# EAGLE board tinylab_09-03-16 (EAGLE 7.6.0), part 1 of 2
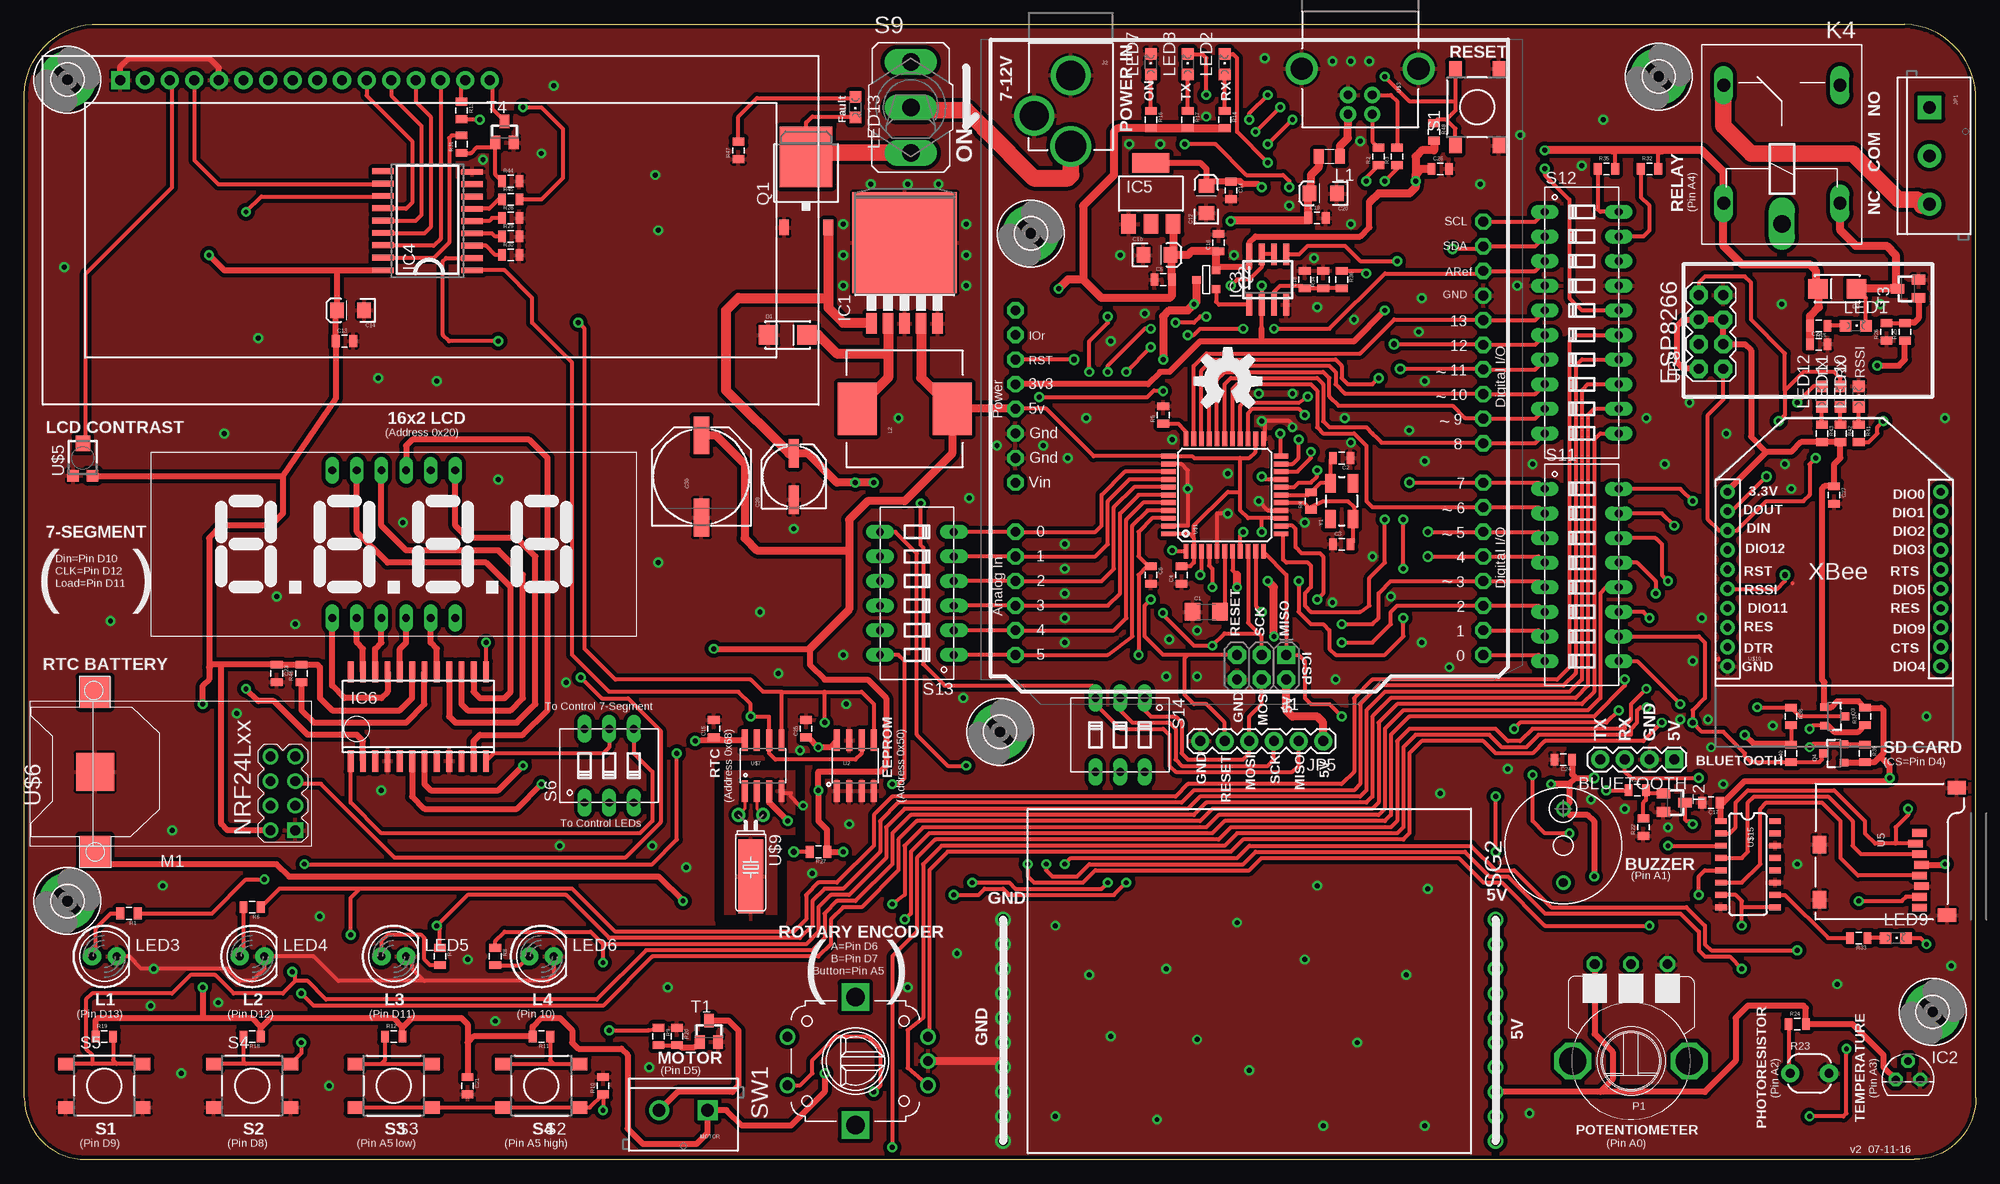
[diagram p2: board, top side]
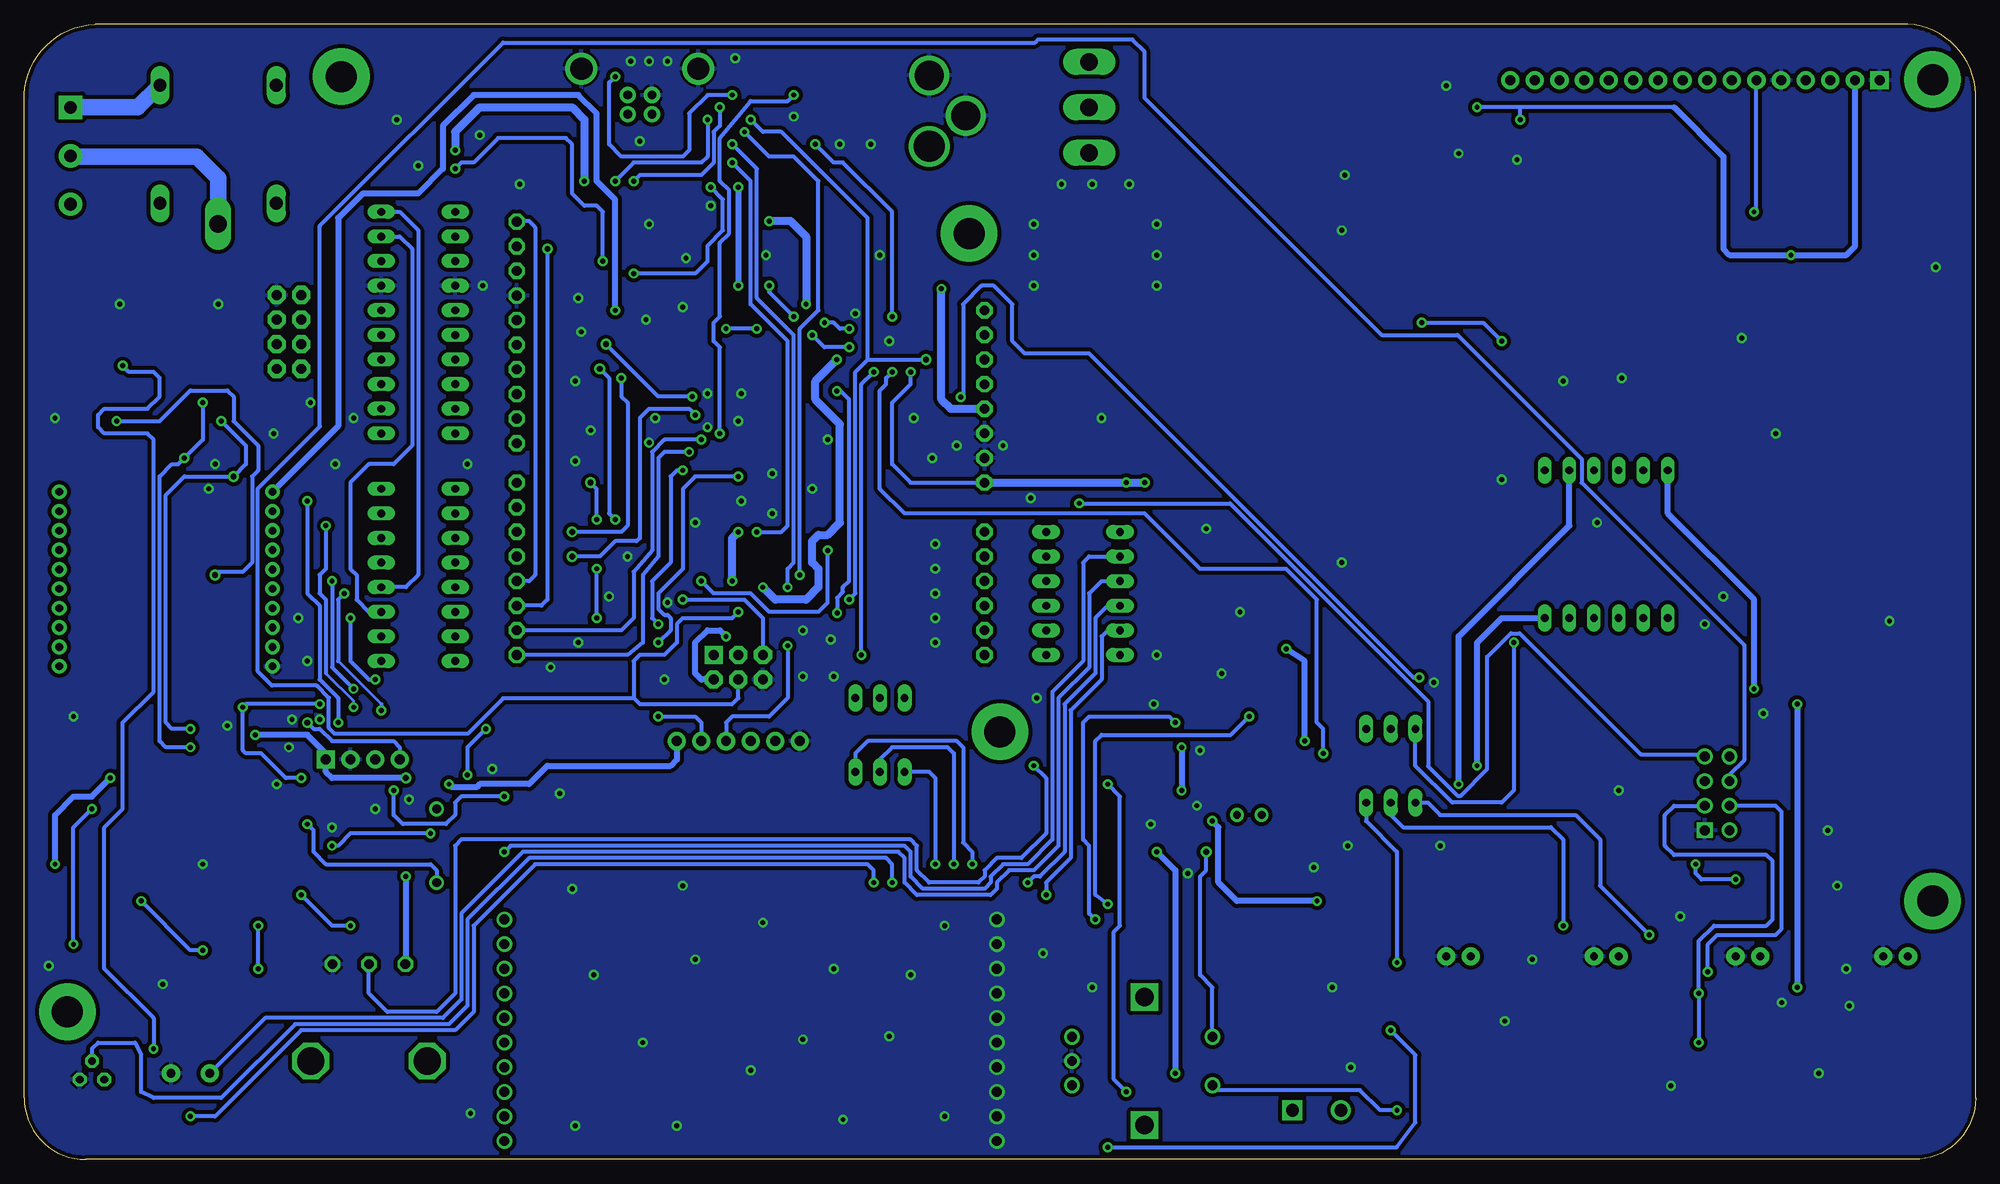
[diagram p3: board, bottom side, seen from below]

Size 201.31 x 117.16 mm. Coordinates in mm from the lower left corner, seen from the top.
Outline: 201.29,6.35 201.29,109.52
Outline: 201.31,6.35 arc-90 194.96,0 6.36,0 arc-90 0.01,6.35 0.01,109.22 arc-90 7,117.16 194,117.16 arc-90 201.31,109.22
Copper layers (1*16): Top 0.035mm / dielectric 1.5mm / Bottom 0.035mm
Design rules "default": minimum track width 16mil, minimum drill 20mil, track to track 8mil, track to pad 12mil, pad to pad 8mil, via to via 8mil, smd to smd 8mil, copper to edge 10mil, drill to drill 8mil, minimum pad ring 12mil, minimum via ring 10mil, stop-mask expansion 4mil, vias tented up to drill 25mil, thermal gap 10mil
tRestrict: 7 lines

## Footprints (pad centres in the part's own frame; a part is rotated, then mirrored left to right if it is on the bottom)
1X04 = drill 1.016 pad 1.88 square: 1 0,0 | drill 1.016 pad 1.88: 2 2.54,0; 3 5.08,0; 4 7.62,0
1206 = smd 1.6 x 1.8: 1 -1.4,0; 2 1.4,0
0805 = smd 0.8 x 1.2: 1 -0.9,0; 2 0.9,0
EIA3216 = smd 1.4 x 1.6: A 1.4,0; C -1.4,0
NIPPON_F80 = smd 2.95 x 1: + 2.4,0; - -2.4,0
PANASONIC_G = smd 3.9 x 1.6: + 4.25,0; - -4.25,0
SMA-DIODE_ALT = smd 2 x 2: A -2,0; C 2,0
3,2-PAD = drill 3.2 pad 5.842: B3,2 0,0
TO263-5 = smd 1.067 x 2.159: 1 -3.404,-5.791; 2 -1.702,-5.791; 3 0,-5.791; 4 1.702,-5.791; 5 3.404,-5.791 | smd 10.8 x 10.41: GND 0,2.54
TO92 = drill 0.813 octagon: 1 -1.27,0; 2 0,1.905; 3 1.27,0
SO08 = smd 0.6 x 2.2: 1 -1.905,-2.6; 2 -0.635,-2.6; 3 0.635,-2.6; 4 1.905,-2.6; 5 1.905,2.6; 6 0.635,2.6; 7 -0.635,2.6; 8 -1.905,2.6
SO18W = smd 0.6 x 2.2: 1 -4.445,-4.6; 2 -3.175,-4.6; 3 -1.905,-4.6; 4 -0.635,-4.6; 5 0.635,-4.6; 6 1.905,-4.6; 7 3.175,-4.6; 8 4.445,-4.6; 9 5.715,-4.6; 10 5.775,4.6; 11 4.505,4.6; 12 3.235,4.6; 13 1.965,4.6; 14 0.695,4.6; 15 -0.575,4.6; 16 -1.845,4.6; 17 -3.145,4.6; 18 -4.445,4.6
SOT223 = smd 1.5 x 2: 1 -2.3,-3.15; 2 0,-3.15; 3 2.3,-3.15 | smd 3.8 x 2: 4 0,3.15
SO24W = smd 0.6 x 2.2: 1 -6.985,-4.6; 2 -5.715,-4.6; 3 -4.445,-4.6; 4 -3.175,-4.6; 5 -1.905,-4.6; 6 -0.635,-4.6; 7 0.635,-4.6; 8 1.905,-4.6; 9 3.175,-4.6; 10 4.445,-4.6; 11 5.715,-4.6; 12 6.985,-4.6; 13 6.985,4.6; 14 5.715,4.6; 15 4.445,4.6; 16 3.175,4.6; 17 1.905,4.6; 18 0.635,4.6; 19 -0.635,4.6; 20 -1.905,4.6; 21 -3.175,4.6; 22 -4.445,4.6; 23 -5.715,4.6; 24 -6.985,4.6
2X3-NS = drill 1.016 pad 1.88 square: 1 -2.54,-1.27 | drill 1.016 pad 1.88 octagon: 2 -2.54,1.27; 3 0,-1.27; 4 0,1.27; 5 2.54,-1.27; 6 2.54,1.27
POWER_JACK_PTH_LOCK = drill 2.997 pad 4.115: GND 0.025,6.557; GNDBREAK 3.762,10.7 | drill 3.2 pad 4.115: PWR 0,13.878
SCREWTERMINAL-5MM-3 = drill 1.3 pad 2.413 square: 1 0,0 | drill 1.3 pad 2.413: 2 5,0; 3 10,0
1X06 = drill 1.016 pad 1.88: 1 0,0; 2 2.54,0; 3 5.08,0; 4 7.62,0; 5 10.16,0; 6 12.7,0
2X4 = drill 1.016 pad 1.88 octagon: 1 -3.81,-1.27; 2 -3.81,1.27; 3 -1.27,-1.27; 4 -1.27,1.27; 5 1.27,-1.27; 6 1.27,1.27; 7 3.81,-1.27; 8 3.81,1.27
ZF112 = drill 1.321 long: 1 -6.096,5.994; 2 -6.096,-5.994; O 6.096,5.994; S 6.096,-5.994 | drill 1.803 long: P -8.204,0
PTC0805 = smd 1 x 1.5: 1 -1.1,0; 2 1.1,0
CDRH125 = smd 5.4 x 4: 1 0,4.9; 2 0,-4.9
CHIPLED_0805 = smd 1.2 x 1.2: A 0,-1.05; C 0,1.05
LED5MM = drill 0.813 pad 1.88: A -1.27,0; K 1.27,0
WIRELESS-NRF24L01 = drill 1 square: 1 -12.7,6.35 | drill 1: 2 -10.16,6.35; 3 -12.7,3.81; 4 -10.16,3.81; 5 -12.7,1.27; 6 -10.16,1.27; 7 -12.7,-1.27; 8 -10.16,-1.27
SCREWTERMINAL-5MM-2 = drill 1.3 pad 2.032 square: 1 0,0 | drill 1.3 pad 2.032: 2 5,0
P120PK = drill 1 octagon: A -3.75,-10; E 3.75,-10; S 0,-10 | drill 2.8 octagon: M1 -6,0; M2 6,0
TO252 = smd 1 x 1.6: 1 -2.28,-4.8; 2 2.28,-4.8 | smd 5.4 x 6.2: 3 0,2.5
SOT-23 = smd 0.787 x 0.889: 1 0.025,-1.016; 2 -0.94,1.016; 3 0.991,1.016
SOT23-3 = smd 0.8 x 0.9: 1 -0.95,-1; 2 0.95,-1; 3 0,1.1
PHOTOCELL-KIT = drill 0.9 pad 1.88: 1 -2,0; 2 2,0
DTSM-6 = smd 1.55 x 1.3: 1 -3.975,2.25; 2 3.975,2.25; 3 -3.975,-2.25; 4 3.975,-2.25
DIP03YL = drill 0.813 long: 1 -2.54,-3.81; 2 0,-3.81; 3 2.54,-3.81; 4 2.54,3.81; 5 0,3.81; 6 -2.54,3.81
M9040P = drill 1.803 long: 1 0,4.699; 2 0,0; 3 0,-4.699
DIP08YL = drill 0.813 long: 1 -8.89,-3.81; 2 -6.35,-3.81; 3 -3.81,-3.81; 4 -1.27,-3.81; 5 1.27,-3.81; 6 3.81,-3.81; 7 6.35,-3.81; 8 8.89,-3.81; 9 8.89,3.81; 10 6.35,3.81; 11 3.81,3.81; 12 1.27,3.81; 13 -1.27,3.81; 14 -3.81,3.81; 15 -6.35,3.81; 16 -8.89,3.81
DIP10YL = drill 0.813 long: 1 -11.43,-3.81; 2 -8.89,-3.81; 3 -6.35,-3.81; 4 -3.81,-3.81; 5 -1.27,-3.81; 6 1.27,-3.81; 7 3.81,-3.81; 8 6.35,-3.81; 9 8.89,-3.81; 10 11.43,-3.81; 11 11.43,3.81; 12 8.89,3.81; 13 6.35,3.81; 14 3.81,3.81; 15 1.27,3.81; 16 -1.27,3.81; 17 -3.81,3.81; 18 -6.35,3.81; 19 -8.89,3.81; 20 -11.43,3.81
DIP06YL = drill 0.813 long: 1 -6.35,-3.81; 2 -3.81,-3.81; 3 -1.27,-3.81; 4 1.27,-3.81; 5 3.81,-3.81; 6 6.35,-3.81; 7 6.35,3.81; 8 3.81,3.81; 9 1.27,3.81; 10 -1.27,3.81; 11 -3.81,3.81; 12 -6.35,3.81
BMT1205XH7.5 = drill 0.9 pad 1.5: + 3.8,0; - -3.8,0
PEC12_INCREMENTAL_ENCODER = drill 1: A -2.5,-7.5; B 2.5,-7.5; C 0,-7.5; P1 -2.5,7; P2 2.5,7 | drill 1.9 square: GND@1 -6.6,0; GND@2 6.6,0
SOT23-BEC = smd 1 x 1.4: B -0.95,-1.1; C 0,1.1; E 0.95,-1.1
LCD-16X2 = drill 1.016 pad 1.88 square: 1 -32,15.5 | drill 1.016 pad 1.88: 2 -29.46,15.5; 3 -26.92,15.5; 4 -24.38,15.5; 5 -21.84,15.5; 6 -19.3,15.5; 7 -16.76,15.5; 8 -14.22,15.5; 9 -11.68,15.5; 10 -9.14,15.5; 11 -6.6,15.5; 12 -4.06,15.5; 13 -1.52,15.5; 14 1.02,15.5; 15 3.56,15.5; 16 6.1,15.5
SO08' = smd 0.61 x 2.21: 1 -1.905,-2.616; 2 -0.635,-2.616; 3 0.635,-2.616; 4 1.905,-2.616; 5 1.905,2.616; 6 0.635,2.616; 7 -0.635,2.616; 8 -1.905,2.616
MICRO-SD-SOCKET-PP = smd 0.8 x 1.5: 1 -8.94,10.7; 2 -7.84,10.3; 3 -6.74,10.7; 4 -5.64,10.9; 5 -4.54,10.7; 6 -3.44,10.9; 7 -2.34,10.7; 8 -1.24,10.7 | smd 1.8 x 1.4: CD1 -2.05,0.4; CD2 -7.75,0.4 | smd 1.4 x 1.9: GND1 -13.6,14.55; GND3 -0.45,13.55
TQFP44 = smd 1.5 x 0.5: 1 -5.8,4; 2 -5.8,3.2; 3 -5.8,2.4; 4 -5.8,1.6; 5 -5.8,0.8; 6 -5.8,0; 7 -5.8,-0.8; 8 -5.8,-1.6; 9 -5.8,-2.4; 10 -5.8,-3.2; 11 -5.8,-4; 23 5.8,-4; 24 5.8,-3.2; 25 5.8,-2.4; 26 5.8,-1.6; 27 5.8,-0.8; 28 5.8,0; 29 5.8,0.8; 30 5.8,1.6; 31 5.8,2.4; 32 5.8,3.2; 33 5.8,4 | smd 0.5 x 1.5: 12 -4,-5.8; 13 -3.2,-5.8; 14 -2.4,-5.8; 15 -1.6,-5.8; 16 -0.8,-5.8; 17 0,-5.8; 18 0.8,-5.8; 19 1.6,-5.8; 20 2.4,-5.8; 21 3.2,-5.8; 22 4,-5.8; 34 4,5.8; 35 3.2,5.8; 36 2.4,5.8; 37 1.6,5.8; 38 0.8,5.8; 39 0,5.8; 40 -0.8,5.8; 41 -1.6,5.8; 42 -2.4,5.8; 43 -3.2,5.8; 44 -4,5.8
USB-B-PTH = drill 0.914 pad 1.676: D+ 0,1.25; D- 1.981,1.25; GND 0,-1.25; VBUS 1.981,-1.25 | drill 2.286: S1 -2.718,-6.02; S2 -2.718,6.02
UNO_R3 = drill 1 pad 1.676 octagon: 3V 35.56,2.54; 5V 38.1,2.54; A0 50.8,2.54; A1 53.34,2.54; A2 55.88,2.54; A3 58.42,2.54; A4 60.96,2.54; A5 63.5,2.54; AREF 23.876,50.8; D0 63.5,50.8; D1 60.96,50.8; D2 58.42,50.8; D3 55.88,50.8; D4 53.34,50.8; D5 50.8,50.8; D6 48.26,50.8; D7 45.72,50.8; D8 41.656,50.8; D9 39.116,50.8; D10 36.576,50.8; D11 34.036,50.8; D12 31.496,50.8; D13 28.956,50.8; GND 26.416,50.8; GND1 43.18,2.54; GND2 40.64,2.54; IOREF 30.48,2.54; RESERVED 27.94,2.54; RESET 33.02,2.54; SCL 18.796,50.8; SDA 21.336,50.8; VIN 45.72,2.54
TC33X = smd 1.2 x 1.2: 1 -1,-1.825; 3 1,-1.825 | smd 1.5 x 1.6: 2 0,1.5
CR1220-SMD = smd 3.2 x 3.2: +$1 -8.2,0; +$2 8.2,0 | smd 3.9 x 3.9: - 0,0
TC38H_GNDPAD = drill 0.813: 1 -1.27,0; 2 1.27,0 | smd 2.54 x 7.62: P$1 0,6.35
XBEE-SILK = drill 0.8 pad 1.524: 1 -11,20; 2 -11,18; 3 -11,16; 4 -11,14; 5 -11,12; 6 -11,10; 7 -11,8; 8 -11,6; 9 -11,4; 10 -11,2; 11 11,2; 12 11,4; 13 11,6; 14 11,8; 15 11,10; 16 11,12; 17 11,14; 18 11,16; 19 11,18; 20 11,20
MYLIB_LDQ_4D_7SEG = drill 0.8 long: 1 -6.35,-7.62; 2 -3.81,-7.62; 3 -1.27,-7.62; 4 1.27,-7.62; 5 3.81,-7.62; 6 6.35,-7.62; 7 6.35,7.62; 8 3.81,7.62; 9 1.27,7.62; 10 -1.27,7.62; 11 -3.81,7.62; 12 -6.35,7.62
SO016 = smd 0.6 x 1.2: 1 -4.445,-2.8; 2 -3.175,-2.8; 3 -1.905,-2.8; 4 -0.635,-2.8; 5 0.635,-2.8; 6 1.905,-2.8; 7 3.175,-2.8; 8 4.445,-2.8; 9 4.445,2.8; 10 3.175,2.8; 11 1.905,2.8; 12 0.635,2.8; 13 -0.635,2.8; 14 -1.905,2.8; 15 -3.175,2.8; 16 -4.445,2.8
CRYSTAL-SMD-5X3 = smd 1.9 x 1.1: 1 -1.85,-1.15; 2 1.85,-1.15; 3 1.85,1.15; 4 -1.85,1.15

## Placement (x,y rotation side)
BLUETOOTH  [1X04]  170.19,41.28 180 top
C1  1uF  [1206]  121.93,56.52 0 top
C2  22pF  [0805]  135.9,72.39 180 top
C3  22pF  [0805]  135.9,63.5 0 top
C4  100nF  [0805]  119.39,60.33 90 top
C5  100nF  [0805]  117.49,90.8 0 top
C6  100nF  [0805]  116.22,60.33 270 top
C10  10uF  [EIA3216]  116.85,93.34 0 top
C11  100nF  [0805]  124.47,100.01 270 top
C12  10uF  [EIA3216]  121.93,99.06 90 top
C13  100nf  [0805]  33.03,84.45 0 top
C14  10uf  [EIA3216]  33.67,87.63 180 top
C15  100nF  [0805]  71.13,44.45 90 top
C16  100nF  [0805]  123.2,94.61 90 top
C17  100nF  [0805]  174,36.83 180 top
C18  100nF  [0805]  132.09,90.8 90 top
C19  100nF  [0805]  133.36,97.16 0 top
C20  10uF  [EIA3216]  134,99.69 180 top
C21  100nF  [0805]  45.73,7.62 270 top
C22  100nF  [0805]  185.11,84.14 0 top
C23  100nf  [0805]  26.05,50.17 270 top
C24  100nF  [0805]  158.76,41.28 180 top
C25  100nF  [0805]  80.66,44.45 90 top
C26  100nF  [0805]  146.06,102.23 0 top
C27  100nF  [0805]  186.7,68.58 270 top
C28  100uF  [NIPPON_F80]  79.39,70.48 90 top
C30  470uF  [PANASONIC_G]  69.86,70.48 90 top
D1  1N4007  [SMA-DIODE_ALT]  78.75,85.09 0 top
D2  1N4007  [SMA-DIODE_ALT]  187.02,89.85 180 top
H1  MOUNT-PAD-ROUND3.2  [3,2-PAD]  4.46,26.67 0 top
H2  MOUNT-PAD-ROUND3.2  [3,2-PAD]  100.66,44.13 0 top
H3  MOUNT-PAD-ROUND3.2  [3,2-PAD]  196.86,15.24 0 top
H4  MOUNT-PAD-ROUND3.2  [3,2-PAD]  168.6,111.76 0 top
H5  MOUNT-PAD-ROUND3.2  [3,2-PAD]  4.46,111.44 0 top
H6  MOUNT-PAD-ROUND3.2  [3,2-PAD]  103.83,95.57 0 top
IC1  LM2575S  [TO263-5]  90.82,92.08 0 top
IC2  LM35CZ  [TO92]  194.32,8.26 0 top
IC3  LM358MX  [SO08]  128.28,90.8 0 top
IC4  MCP2300X/SO  [SO18W]  41.6,96.2 90 top
IC5  LD117AS33TR  [SOT223]  116.22,99.69 0 top
IC6  MAX7219CWG  [SO24W]  40.65,45.72 0 top
J1  AVR_SPI_PRG_6NS  [2X3-NS]  127.65,50.8 180 top
J2  POWER_JACKPTH_LOCK  [POWER_JACK_PTH_LOCK]  107.96,118.43 180 top
JP1  [SCREWTERMINAL-5MM-3]  196.54,108.58 270 top
JP5  [1X06]  134,43.18 180 top
JP8  [2X4]  174,85.41 90 top
K4  ZF112  [ZF112]  181.3,104.77 90 top
L1  [PTC0805]  134.63,103.5 180 top
L2  [CDRH125]  90.82,77.47 90 top
LED1  Blue  [CHIPLED_0805]  188.92,86.04 270 top
LED2  Green  [CHIPLED_0805]  123.84,113.03 0 top
LED3  RED  [LED5MM]  8.27,20.95 0 top
LED4  RED  [LED5MM]  23.51,20.95 0 top
LED5  RED  [LED5MM]  38.11,20.95 0 top
LED6  RED  [LED5MM]  53.35,20.95 0 top
LED7  Yellow  [CHIPLED_0805]  116.22,113.03 0 top
LED8  Green  [CHIPLED_0805]  120.03,113.03 0 top
LED9  Blue  [CHIPLED_0805]  193.05,22.86 270 top
LED10  Yellow  [CHIPLED_0805]  189.24,78.74 0 top
LED11  Red  [CHIPLED_0805]  187.34,78.74 0 top
LED12  Blue  [CHIPLED_0805]  185.43,78.74 0 top
LED13  Red  [CHIPLED_0805]  85.74,108.58 180 top
M1  WIRELESS-NRF24L01  [WIRELESS-NRF24L01]  15.25,40.32 180 top
MOTOR  [SCREWTERMINAL-5MM-2]  70.5,5.08 180 top
P1  P120PK  [P120PK]  165.75,10.16 180 top
Q1  FDD4141 or FDD6637  [TO252]  80.66,100.96 0 top
Q2  FDN340  [SOT-23]  121.93,90.8 270 top
Q3  BSS138  [SOT23-3]  186.7,45.72 270 top
Q4  BSS138  [SOT23-3]  186.7,41.91 90 top
R1  330  [0805]  10.81,25.4 180 top
R2  22  [0805]  139.71,103.5 90 top
R3  22  [0805]  141.62,103.5 90 top
R4  1M  [0805]  132.73,67.94 90 top
R5  10K  [0805]  117.49,76.83 90 top
R6  330  [0805]  23.51,26.04 180 top
R7  330  [0805]  42.87,20.95 270 top
R8  330  [0805]  48.59,20.95 270 top
R9  1k  [0805]  65.42,12.7 270 top
R10  1k  [0805]  59.7,7.62 90 top
R11  1k  [0805]  53.35,12.7 180 top
R12  3.9k  [0805]  38.11,12.7 0 top
R13  100R  [0805]  45.1,108.27 270 top
R14  330  [0805]  123.84,107.31 270 top
R15  1k  [0805]  185.11,86.04 180 top
R16  330  [0805]  116.22,107.31 270 top
R17  330  [0805]  120.03,107.31 270 top
R18  10k  [0805]  23.51,12.7 180 top
R19  10k  [0805]  8.27,12.7 0 top
R20  10k  [0805]  67.32,12.7 270 top
R21  1k  [0805]  166.38,38.1 0 top
R22  10k  [0805]  167.02,34.29 90 top
R23  PHOTOCELLPTH-KIT  [PHOTOCELL-KIT]  184.16,8.89 0 top
R24  10k  [0805]  182.89,13.97 0 top
R25  1k  [0805]  194,85.41 90 top
R26  10k  [0805]  192.1,85.41 90 top
R27  10k  [0805]  81.93,31.75 180 top
R28  10k  [0805]  50.18,97.16 0 top
R29  10k  [0805]  50.18,95.25 0 top
R30  10k  [0805]  50.18,93.34 0 top
R31  1k  [0805]  45.1,104.77 90 top
R32  4.7k  [0805]  167.65,102.23 0 top
R33  1k  [0805]  189.24,22.86 180 top
R34  10K  [0805]  134,90.8 90 top
R35  4.7k  [0805]  163.21,102.23 0 top
R36  10K  [0805]  135.9,90.8 270 top
R37  10K  [0805]  189.88,45.72 90 top
R38  10K  [0805]  182.26,45.72 270 top
R39  10K  [0805]  189.88,41.91 270 top
R40  10K  [0805]  182.26,41.91 90 top
R41  1K  [0805]  189.24,74.93 270 top
R42  1K  [0805]  187.34,74.93 270 top
R43  1K  [0805]  185.43,74.93 270 top
R44  10k  [0805]  50.18,100.96 0 top
R45  10k  [0805]  50.18,99.06 0 top
R46  30k  [0805]  28.59,50.17 90 top
R47  1k  [0805]  73.67,104.14 90 top
R48  10k  [0805]  145.43,106.05 270 top
S1  DTSM-6  [DTSM-6]  149.87,108.58 90 top
S2  DTSM-6  [DTSM-6]  53.35,7.62 180 top
S3  DTSM-6  [DTSM-6]  38.11,7.62 180 top
S4  DTSM-6  [DTSM-6]  23.51,7.62 0 top
S5  DTSM-6  [DTSM-6]  8.27,7.62 0 top
S6  [DIP03YL]  60.34,40.64 0 top
S9  [M9040P]  91.45,108.58 0 top
S11  [DIP08YL]  160.67,60.33 270 top
S12  [DIP10YL]  160.67,86.36 270 top
S13  [DIP06YL]  92.09,58.42 90 top
S14  [DIP03YL]  113.04,43.82 180 top
SG2  BMT1205XH7.5  [BMT1205XH7.5]  158.76,32.38 90 top
SW1  ENCODER_SW1-PEC12  [PEC12_INCREMENTAL_ENCODER]  85.74,10.16 90 top
T1  BC847  [SOT23-BEC]  70.62,13.23 0 top
T2  BC847  [SOT23-BEC]  170.19,36.83 270 top
T3  BC847  [SOT23-BEC]  194.32,89.85 90 top
T4  BC847  [SOT23-BEC]  49.54,106.05 0 top
U1  LCD-16X2SILK  [LCD-16X2]  41.92,95.88 0 top
U2  24LC256  [SO08']  85.74,40.64 0 top
U5  USD-SOCKETNEW  [MICRO-SD-SOCKET-PP]  184.8,24.77 270 top
U$1  ATMEGA32U4TQFP-44  [TQFP44]  123.84,68.58 90 top
U$2  BREADBOARDMINI  [BREADBOARD-MINI]  149.24,36.2 180 top
U$3  USB+SHIELD  [USB-B-PTH]  137.81,109.85 270 top
U$4  UNO_R3  [UNO_R3]  99.71,115.57 270 top
U$5  10k  [TC33X]  6.04,72.39 0 top
U$6  [CR1220-SMD]  7.31,40.01 90 top
U$7  DS1307SO8  [SO08']  76.21,40.64 0 top
U$9  CRYSTAL_GNDPAD  [TC38H_GNDPAD]  74.94,35.56 180 top
U$10  XBEE-1B2  [XBEE-SILK]  186.7,48.9 0 top
U$11  [TINYLAB_LOGO_LARGE]  31.13,22.54 0 top
U$13  MYLIB_LCQ_4D_7SEG  [MYLIB_LDQ_4D_7SEG]  38.11,63.5 0 top
U$14  [OSHW-LOGO-L]  124.15,80.33 0 top
U$15  74HC4050  [SO016]  177.81,30.48 270 top
Y1  16Mhz  [CRYSTAL-SMD-5X3]  135.9,67.94 90 top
